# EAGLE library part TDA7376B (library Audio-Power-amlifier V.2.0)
The TDA7376B is a new technology dual bridge Audio Amplifier in Multiwatt 15 package designed for car radio applications. Thanks to the fully complementary PNP/NPN output stage configuration the TDA7376B delivers a rail-to-rail voltage swing with no need of bootstrap capacitors. Differential input pairs, that will accept either single ended or differential input signals, guarantee high noise immunity making the device suitable for both car radio and car boosters applications.
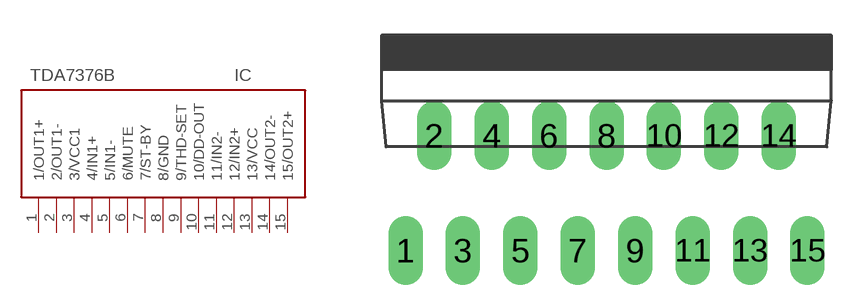
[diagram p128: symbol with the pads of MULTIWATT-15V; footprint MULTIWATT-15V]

Designator prefix IC

## TDA7376B  [MULTIWATT-15V]
1  1/OUT1+  out
2  2/OUT1-  out
3  3/VCC1  pwr
4  4/IN1+  in
5  5/IN1-  in
6  6/MUTE  in
7  7/ST-BY  in
8  8/GND  pwr
9  9/THD-SET
10  10/DD-OUT  out
11  11/IN2-  in
12  12/IN2+  pwr
13  13/VCC  out
14  14/OUT2-  out
15  15/OUT2+  out

## Footprint MULTIWATT-15V (pad centres in mm)
Multiwatt 15 vertical
drill 1.016 long: 1 -8.89,-5.08; 2 -7.62,0; 3 -6.35,-5.08; 4 -5.08,0; 5 -3.81,-5.08; 6 -2.54,0; 7 -1.27,-5.08; 8 0,0; 9 1.27,-5.08; 10 2.54,0; 11 3.81,-5.08; 12 5.08,0; 13 6.35,-5.08; 14 7.62,0; 15 8.89,-5.08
